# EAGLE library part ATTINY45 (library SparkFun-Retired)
Atmel 8-pin 2/4/8kB flash uC Retired
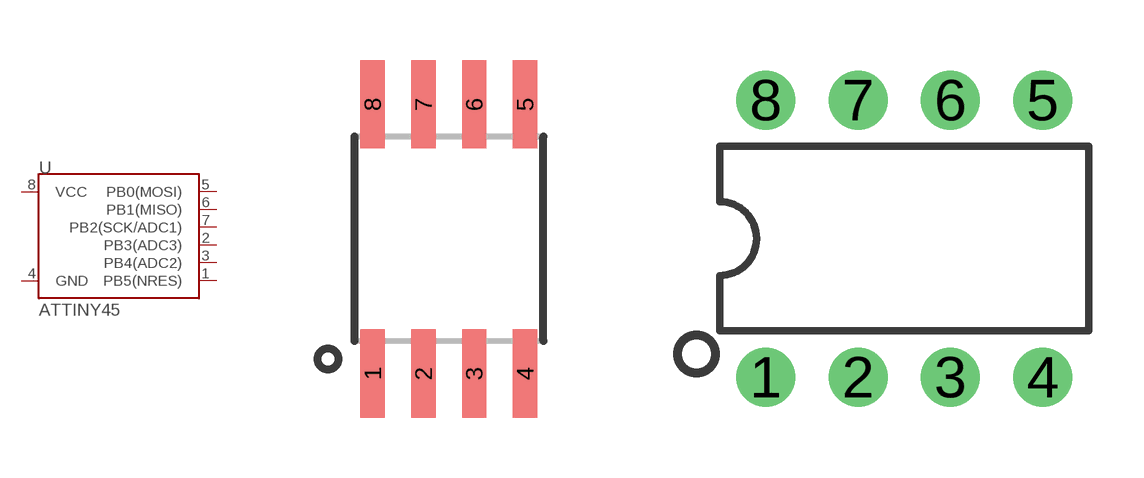
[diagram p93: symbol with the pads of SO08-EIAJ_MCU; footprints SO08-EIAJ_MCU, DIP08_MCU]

Designator prefix U

## ATTINY45TINY45-20-SMT (PROD_ID: IC-08922; VALUE: Tiny45-20-SMT)  [SO08-EIAJ_MCU]
1  PB5(NRES)
2  PB3(ADC3)
3  PB4(ADC2)
4  GND
5  PB0(MOSI)
6  PB1(MISO)
7  PB2(SCK/ADC1)
8  VCC

## ATTINY45TINY45-20-DIP (PROD_ID: IC-09439; VALUE: TINY45-20-DIP)  [DIP08_MCU]
Pads as for SO08-EIAJ_MCU

## ATTINY45TINY85-20-DIP (PROD_ID: IC-09445; VALUE: TINY85-20-DIP)  [DIP08_MCU]
Pads as for SO08-EIAJ_MCU

## ATTINY45TINY85-20-SMT (PROD_ID: IC-09092; VALUE: Tiny85-20-SMT)  [SO08-EIAJ_MCU]
Pads as for SO08-EIAJ_MCU

## Footprint SO08-EIAJ_MCU (pad centres in mm)
Fits EIAJ packages (wide version of the SOIC-8).
smd 0.61 x 2.21: 1 -1.905,-3.378; 2 -0.635,-3.378; 3 0.635,-3.378; 4 1.905,-3.378; 5 1.905,3.353; 6 0.635,3.353; 7 -0.635,3.353; 8 -1.905,3.353

## Footprint DIP08_MCU (pad centres in mm)
Dual In Line Package
drill 0.813 pad 1.626: 1 -3.81,-3.81; 2 -1.27,-3.81; 3 1.27,-3.81; 4 3.81,-3.81; 5 3.81,3.81; 6 1.27,3.81; 7 -1.27,3.81; 8 -3.81,3.81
